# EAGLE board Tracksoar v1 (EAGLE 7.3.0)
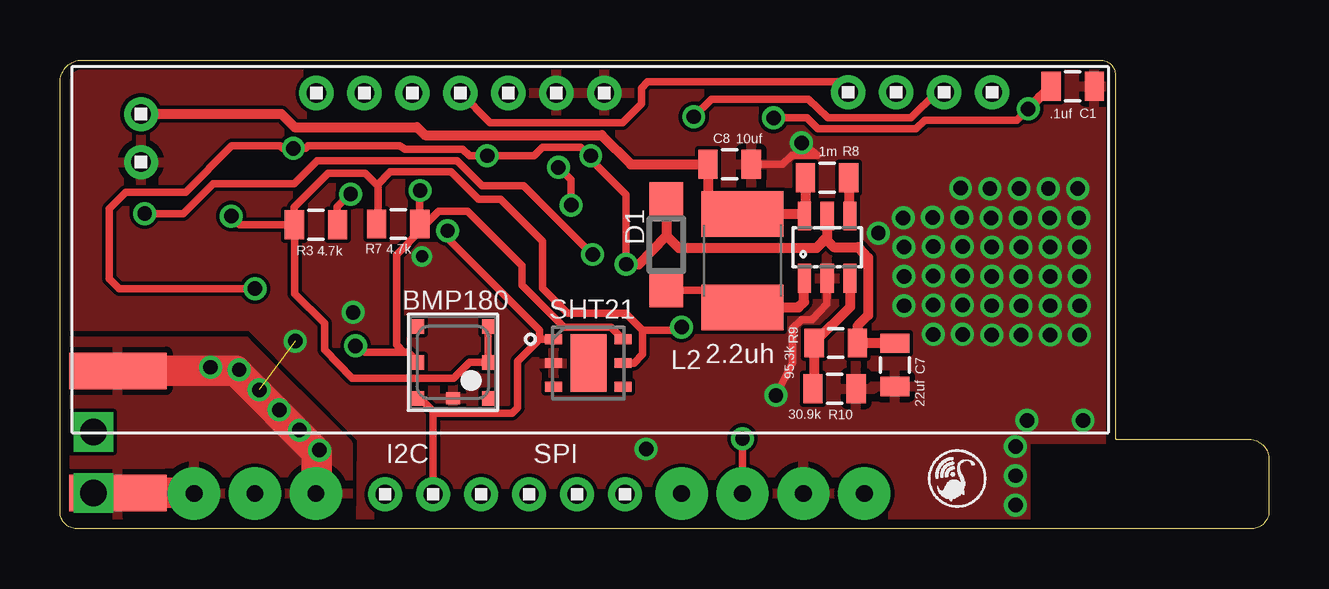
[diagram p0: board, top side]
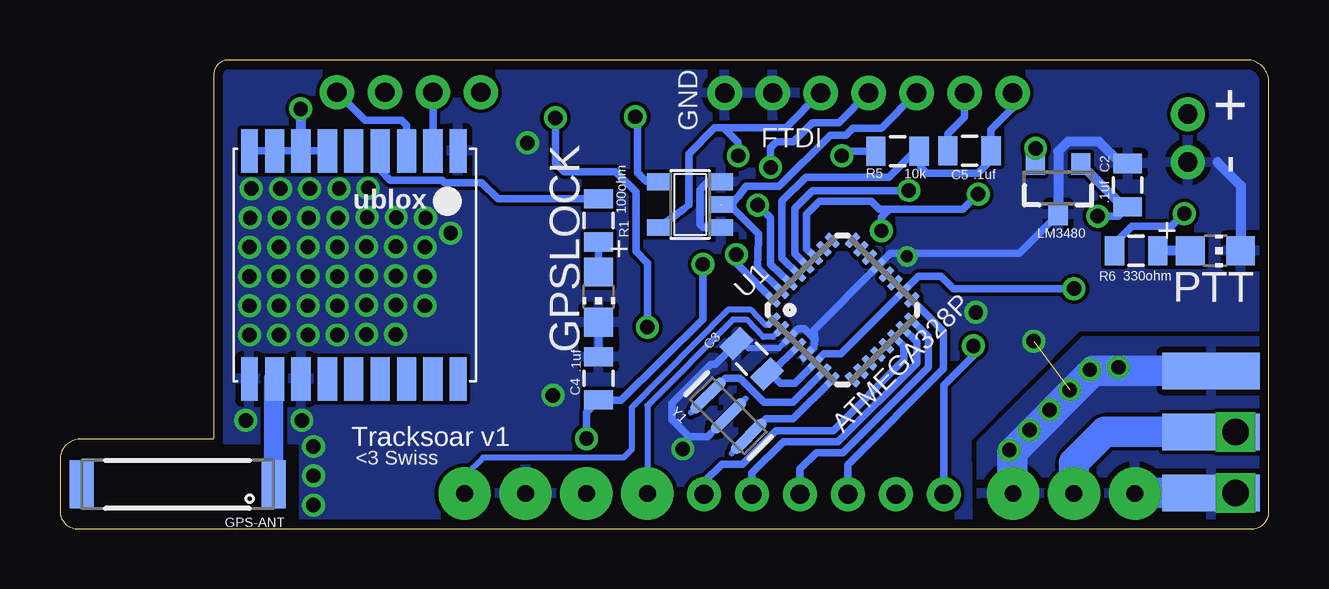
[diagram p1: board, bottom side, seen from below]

Size 50.39 x 19.53 mm. Coordinates in mm from the lower left corner, seen from the top.
Outline: 0.69,0 arc-90 0,0.76 0,18.67 arc-90 0.99,19.53 43.38,19.53 arc-90 43.99,18.87 43.99,3.78 arc90 44.04,3.73 49.58,3.73 arc-90 50.39,2.87 50.39,0.79 arc-90 49.68,0 0.69,0
Copper layers (1*16): Top 0.0356mm / dielectric 1.5011mm / Bottom 0.0356mm
Design rules "oshpark-2layer": minimum track width 6mil, minimum drill 13mil, track to track 6mil, track to pad 6mil, pad to pad 6mil, via to via 6mil, smd to smd 6mil, copper to edge 15mil, drill to drill 6mil, minimum pad ring 7mil, minimum via ring 7mil, stop-mask expansion 4mil, vias tented up to drill 0mil, thermal gap 10mil

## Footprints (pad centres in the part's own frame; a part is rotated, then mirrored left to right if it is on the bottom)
BMP180 = smd 0.6 x 0.5: 1 1.5,1.45; 2 0,1.45; 3 -1.5,1.45; 4 -1.5,-1.45; 5 0,-1.45; 6 1.5,-1.45 | smd 0.5 x 0.6: 7 1.5,0
0805 = smd 0.8 x 1.2: 1 -0.9,0; 2 0.9,0
SOD123 = smd 1.4 x 1.4: A 1.9,0; C -1.9,0
1X7 = drill 0.8 pad 1.422: 1 -6,0; 2 -4,0; 3 -2,0; 4 0,0; 5 2,0; 6 4,0; 7 6,0
ANTENNA-CHIP4 = smd 1 x 2: NC 4,0; SIG -4,0
CHIP-LED0805 = smd 1.2 x 1.2: A 0,-1.05; C 0,1.05
SOT23-5 = smd 0.69 x 0.99: 1 -0.95,-1.29; 2 0,-1.29; 3 0.95,-1.29; 4 0.95,1.3; 5 -0.95,1.3
SMA-EDGE = smd 1.524 x 4.064: GND@0 0,0; GND@1 5.08,0; SIG 2.54,0 | smd 1.524 x 4.064 bottom: GND@2 0,0; GND@3 5.08,0
L1812 = smd 1.9 x 3.4: 1 -1.95,0; 2 1.95,0
SOT23-3 = smd 0.8 x 0.9: 1 -0.95,-1; 2 0.95,-1; 3 0,1.1
SOT23-6 = smd 0.55 x 1.2: 1 -0.95,-1.3; 2 0,-1.3; 3 0.95,-1.3; 4 0.95,1.3; 5 0,1.3; 6 -0.95,1.3
1X4 = drill 0.8 pad 1.422: 1 -3,0; 2 -1,0; 3 1,0; 4 3,0
DFN300X300X110-7N = smd 0.711 x 0.406: 1 -1.448,0.991; 2 -1.448,0; 3 -1.448,-0.991; 4 1.448,-0.991; 5 1.448,0; 6 1.448,0.991 | smd 1.499 x 2.388: 7 0,0
1X6 = drill 0.8 pad 1.422: 1 -5,0; 2 -3,0; 3 -1,0; 4 1,0; 5 3,0; 6 5,0
MLF32 = smd 0.7 x 0.3: 1 -2.35,1.75; 2 -2.35,1.25; 3 -2.35,0.75; 4 -2.35,0.25; 5 -2.35,-0.25; 6 -2.35,-0.75; 7 -2.35,-1.25; 8 -2.35,-1.75; 17 2.35,-1.75; 18 2.35,-1.25; 19 2.35,-0.75; 20 2.35,-0.25; 21 2.35,0.25; 22 2.35,0.75; 23 2.35,1.25; 24 2.35,1.75 | smd 0.3 x 0.7: 9 -1.75,-2.35; 10 -1.25,-2.35; 11 -0.75,-2.35; 12 -0.25,-2.35; 13 0.25,-2.35; 14 0.75,-2.35; 15 1.25,-2.35; 16 1.75,-2.35; 25 1.75,2.35; 26 1.25,2.35; 27 0.75,2.35; 28 0.25,2.35; 29 -0.25,2.35; 30 -0.75,2.35; 31 -1.25,2.35; 32 -1.75,2.35
UBLOX_MAX = smd 1.8 x 0.7: 1_GND 4.95,-4.4; 9_V_RESET 4.95,4.3; 10_GND -4.55,4.3; 18_RESERVED -4.55,-4.4 | smd 1.8 x 0.8: 2_TXD1 4.95,-3.35; 3_RXD1 4.95,-2.25; 4_TIMEPULSE 4.95,-1.15; 5_EXTINT0 4.95,-0.05; 6_V_BCKP 4.95,1.05; 7_VCC_IO 4.95,2.15; 8_VCC 4.95,3.25; 11_RF_IN -4.55,3.25; 12_GND -4.55,2.15; 13_ANTON -4.55,1.05; 14_VCC_RF -4.55,-0.05; 15_RESERVED -4.55,-1.15; 16_SDA2 -4.55,-2.25; 17_SCL2 -4.55,-3.35
RADIOMETRIX-HX1 = drill 0.7 pad 2.184: 0V 8.89,-10.16; EN 3.81,-10.16; RFGND -11.43,-10.16; RFGND2 -16.51,-10.16; RFOUT -13.97,-10.16; TXD 11.43,-10.16; VCC 6.35,-10.16
1X2 = drill 0.8 pad 1.422: 1 -1,0; 2 1,0
RESONATOR-SMD = smd 0.45 x 1.905: 1 -1.2,0; 2 0,0; 3 1.2,0

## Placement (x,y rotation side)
BMP180  BMP180  [BMP180]  16.38,6.93 270 top
C1  .1uf  [0805]  42.22,18.44 180 top
C2  .1uf  [0805]  5.89,14.33 270 bottom
C3  .1uf  [0805]  21.57,7.09 315 bottom
C4  .1uf  [0805]  27.94,6.27 270 bottom
C5  .1uf  [0805]  12.48,15.76 0 bottom
C7  22uf  [0805]  34.8,6.83 270 top
C8  10uf  [0805]  27.92,15.19 0 top
D1  MBR120VLSFT1  [SOD123]  25.27,11.84 270 top
FRAME1  FRAME-LETTER  [CREATIVE_COMMONS]  not placed on the board
FTDI  1X7  [1X7]  16.69,18.16 180 top
GPS-ANT  ANTENNA2SMD3  [ANTENNA-CHIP4]  45.49,1.85 180 bottom
GPSLOCK  [CHIP-LED0805]  27.94,9.65 180 bottom
IC2  74AHC1G125DBV  [SOT23-5]  24.13,13.51 90 bottom
J$1  SMA_EDGE  [SMA-EDGE]  2.41,1.5 90 bottom
L2  2.2uh  [L1812]  28.45,11.18 270 top
LM3480  LM3480IM4  [SOT23-3]  8.79,14.2 180 bottom
LT3426  LT3426  [SOT23-6]  31.98,11.73 0 top
PTT  [CHIP-LED0805]  2.24,11.58 270 bottom
R1  100ohm  [0805]  27.94,12.85 270 bottom
R3  4.7k  [0805]  10.67,12.67 0 top
R5  10k  [0805]  15.48,15.74 180 bottom
R6  330ohm  [0805]  5.54,11.58 180 bottom
R7  4.7k  [0805]  14.1,12.7 0 top
R8  1m  [0805]  31.98,14.63 180 top
R9  95.3k  [0805]  32.33,7.75 0 top
R10  30.9k  [0805]  32.28,5.84 180 top
SERIAL  1X4  [1X4]  35.86,18.19 180 top
SHT21  SHT21  [DFN300X300X110-7N]  22.02,6.91 0 top
SPI/I2C  1X6  [1X6]  18.56,1.43 0 top
U1  ATMEGA328P  [MLF32]  17.78,9.12 45 bottom
U$1  UBLOX_MAX  [UBLOX_MAX]  38.2,10.79 90 bottom
U$2  RADIOMETRIX-HX1  [RADIOMETRIX-HX1]  22.1,11.63 0 top
U$3  1X2  [1X2]  3.38,16.28 90 top
Y1  16MHZ  [RESONATOR-SMD]  22.53,4.71 315 bottom

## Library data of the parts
BMP180 = SparkFun-Sensors
C1-C5 C7 C8 = SparkFun-Capacitors
D1 = diode
FRAME1 = SparkFun-Aesthetics
FTDI SERIAL SPI/I2C U$3 = headers(2mm)
GPS-ANT = SparkFun-RF
GPSLOCK LT3426 PTT = adafruit
IC2 = 74xx-little-us
J$1 = SparkFun-Connectors
L2 = resistor
LM3480 = SparkFun-PowerIC
R1 R3 R5-R10 = SparkFun-Resistors
SHT21 = sht21; MPN: SHT21; OC_FARNELL: 1855468; OC_NEWARK: 20T1172; PACKAGE: DFN-6; SUPPLIER: SENSIRION
U1 = SparkFun-DigitalIC
U$1 U$2 = Ava
Y1 = SparkFun-FreqCtrl; PROD_ID: XTAL-08900

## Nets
3V: BMP180.2 BMP180.3 C1.2 C2.2 LM3480.1 R3.1 R7.1 SHT21.5 U$1.6_V_BCKP U$1.7_VCC_IO U$1.8_VCC U$1.9_V_RESET
15V: C8.1 L2.1 LT3426.6 R8.2 U$3.2
!RESET: C5.2 FTDI.7 R5.1 U1.29
D3: U1.1 U$2.TXD
D4: U1.2 U$2.EN
DTR: C5.1 FTDI.6
GND: BMP180.7 C1.1 C2.1 C3.1 C4.1 C7.2 C8.2 FTDI.1 FTDI.2 GPSLOCK.C IC2.1 IC2.3 J$1.GND@0 J$1.GND@1 J$1.GND@2 J$1.GND@3 LM3480.3 LT3426.2 PTT.C R10.1 SHT21.2 U1.3 U1.5 U1.21 U$1.1_GND U$1.10_GND U$1.12_GND U$2.0V U$2.RFGND U$2.RFGND2 U$3.1 Y1.2
LED: R6.2 U1.32
MISO: SPI/I2C.4 U1.16
MOSI: SPI/I2C.5 U1.15
N$1: J$1.SIG U$2.RFOUT
N$3: GPSLOCK.A R1.2
N$6: GPS-ANT.SIG U$1.11_RF_IN
N$9: D1.A L2.2 LT3426.1
N$12: LT3426.4 R8.1
N$13: LT3426.3 R9.1 R10.2
N$14: U1.8 Y1.3
N$26: U1.7 Y1.1
N$27: PTT.A R6.1
PPS: R1.1 U$1.4_TIMEPULSE
RX1: SERIAL.1 U$1.3_RXD1
RXO: FTDI.4 SERIAL.4 U1.30
SCK: SPI/I2C.3 U1.17
SCL: BMP180.5 R7.2 SHT21.6 SPI/I2C.1 U1.28
SDA: BMP180.6 R3.2 SHT21.1 SPI/I2C.2 U1.27
SS: SPI/I2C.6 U1.14
TX: SERIAL.3 U$1.2_TXD1
TX1: IC2.4 SERIAL.2
TXO: FTDI.5 IC2.2 U1.31
VCC: C3.2 C4.2 C7.1 D1.C FTDI.3 IC2.5 LM3480.2 LT3426.5 R5.2 R9.2 U1.4 U1.6 U1.18 U$2.VCC

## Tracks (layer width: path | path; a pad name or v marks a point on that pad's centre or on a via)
3V  (via drill 0.6)
  Top 0.305: R3.1 7.49,12.67 v7.14,13.03 | R3.1 9.77,13.4 11.18,14.81 12.73,14.81 13.21,14.33 | 13.21,14.33 13.26,14.21 13.26,12.76 R7.1 | 13.21,14.33 13.77,14.88 16.31,14.88 17.45,13.74 18.37,13.74 20.12,11.99 20.12,10.03 21.16,8.99 23.57,8.99 24.28,8.28 | R3.1 9.78,12.66 9.78,9.8 11.02,8.56 11.02,7.47 12.17,6.27 16.41,6.27 17.07,6.93 BMP180.2 BMP180.3 | SHT21.5 23.93,6.91 24.28,7.26 24.28,8.28 | 40.89,17.99 C1.2 | 24.28,8.28 25.78,8.28 v25.91,8.41 | v40.36,17.5 39.88,17.02 36.04,17.02 35.69,16.66 31.6,16.66 31.14,17.12 v29.74,17.12
  Top 0.406: C1.2 40.84,17.98 v40.36,17.5
  Bottom 0.305: U$1.9_V_RESET U$1.8_VCC U$1.7_VCC_IO U$1.6_V_BCKP 39.27,15.73 | v7.14,13.03 6.29,13.03 C2.2 | v25.91,8.41 25.91,11.07 26.39,11.56 26.39,14.05 27.23,14.88 29.39,14.88 29.74,15.24 v29.74,17.12
  Bottom 0.406: C2.2 6.07,13.43 LM3480.1 | v40.36,17.5 U$1.7_VCC_IO
15V
  Top 0.406: U$3.2 9.24,17.28 9.78,16.74 14.89,16.74 15.22,16.41 22.58,16.41 23.8,15.19 C8.1 27.02,13.85 27.76,13.11 28.43,13.11 L2.1 30.94,13.13 LT3426.6 31.08,13.08 R8.2
!RESET
  Bottom 0.305: U1.29 20.3,11.28 20.3,13.67 19.3,14.66 15.85,14.66 14.77,15.74 R5.1 14.5,15.06 14.25,14.81 12.14,14.81 11.58,15.37 C5.2 11.58,16.64 10.69,17.53 FTDI.7
D3
  Bottom 0.254: U1.1 20.89,8.48 20.98,8.48 21.59,9.12 22.56,9.12 26.57,5.05 26.57,3.3 26.9,2.97 32.77,2.97 33.53,2.21 U$2.TXD
D4
  Bottom 0.254: U1.2 20.67,8 21.08,8 21.77,8.71 22.35,8.71 25.91,5.13 U$2.EN
DTR
  Bottom 0.305: FTDI.6 12.69,17.16 13.39,16.46 13.39,15.77
  Bottom 0.406: 13.39,15.77 C5.1
GND  (via drill 0.5, 0.6, 1.1)  (1 unrouted)
  Top 0.305: LT3426.2 31.98,9.37 31.34,8.71 30.91,8.71 30.53,8.36 30.53,6.91 v29.85,5.56 | C8.2 30.13,15.19 30.51,15.57 31.57,15.57 v30.91,16.08
  Top 0.406: U$2.RFGND2 5.61,1.47 5.61,1.5
  Top 1.27: J$1.GND@1 7.32,6.58 10.69,3.2 10.69,1.5 U$2.RFGND | 2.31,1.5 5.61,1.5
  Bottom 0.254: U1.3 20.44,7.52 21.69,7.52 21.9,7.72 C3.1
  Bottom 0.305: U1.5 18.97,7.57 18.92,7.9 | 18.92,7.9 19.36,8.33 19.63,8.33 U1.3 | 18.92,7.9 18.97,8.28 U1.21 15.77,11.48 10.41,11.48 LM3480.3 | GPSLOCK.C C4.1 | 22.85,14.49 IC2.3 22.85,14.45 23.39,14.45 23.72,14.12 23.72,12.7 23.59,12.56 IC2.1 | C3.1 23.07,6.86 23.27,6.86 24.89,5.23 24.89,4.55 24.18,3.84 23.41,3.84 23.25,3.99
  Bottom 0.406: 2.15,15.28 1.17,14.3 1.17,11.6 PTT.C | 5.84,15.28 C2.1 6.18,15.23 7.09,16.13 8.38,16.13 8.79,15.72 LM3480.3
  Bottom 1.27: U$2.RFGND2 5.56,1.5 J$1.GND@2 | J$1.GND@1 7.32,6.58 10.69,3.2 10.69,1.5 U$2.RFGND
  other vias: 9.8,7.82 15.09,11.35 12.22,9.02 1.4,1.5 24.44,3.33 42.49,8.08 41.28,8.08 40.06,8.08 38.84,8.08 37.62,8.1 36.4,8.1 42.49,9.3 41.28,9.3 40.06,9.3 38.84,9.3 37.62,9.32 36.4,9.32 35.18,9.3 42.49,10.52 41.28,10.52 40.06,10.52 38.84,10.52 37.62,10.54 36.4,10.54 35.18,10.52 42.49,11.73 41.28,11.73 40.06,11.73 38.84,11.73 37.62,11.76 36.4,11.76 35.18,11.73 42.47,12.95 41.25,12.95 40.03,12.95 38.81,12.95 41.2,14.17 42.65,4.52 39.83,3.43 39.83,2.21 39.83,0.99 40.31,4.52 39.98,14.17 42.42,14.17 37.59,12.98 36.37,12.98 35.15,12.95 34.11,12.32 38.76,14.17 37.54,14.2 6.27,6.73 7.47,6.63 8.31,5.79 9.14,4.95 9.98,4.11 10.82,3.28
  pour Top: 0,19.56 44.02,19.56 44.02,3.73 40.23,3.73 40.23,0 12.55,0 12.6,3.76 7.95,8.43 0,8.43
  pour Bottom: 0,19.56 44.02,19.56 44.02,3.73 40.23,3.73 40.23,0 12.55,0 12.6,3.76 7.95,8.43 0,8.43
  pour Bottom: 0,7.82 7.72,7.82 11.99,3.56 11.99,0 0,0
  pour Top: 0,7.82 7.72,7.82 11.99,3.56 11.99,0 0,0
LED  (via drill 0.6)
  Top 0.305: v3.53,13.13 5.13,13.13 6.38,14.38 9.75,14.38 10.72,15.34 16.56,15.34 17.6,14.3 19.33,14.3 v22.2,11.43
  Bottom 0.305: R6.2 6.44,11.88 5.72,12.6 4.06,12.6 v3.53,13.13 | v22.2,11.43 22.2,11.06 U1.32
MISO
  Bottom 0.305: U1.16 14.2,8.01 14.2,6.73 17.76,3.17 18.87,3.17 19.55,2.5 SPI/I2C.4
MOSI
  Bottom 0.305: U1.15 14.68,7.79 14.68,6.91 17.96,3.63 20.24,3.63 21.55,2.33 SPI/I2C.5
N$1
  Bottom 1.27: J$1.SIG 6.83,4.04 8.13,2.74 U$2.RFOUT
N$3
  Bottom 0.305: R1.2 GPSLOCK.A
N$6
  Bottom 0.813: U$1.11_RF_IN 41.49,6.24 GPS-ANT.SIG
N$9
  Top 0.305: D1.A 27.74,9.94 L2.2
  Top 0.406: L2.2 30.79,9.23 31.01,9.45 31.01,10.42 LT3426.1
N$12
  Top 0.406: R8.1 32.88,13.08 LT3426.4
N$13
  Top 0.406: LT3426.3 32.93,9.24 R9.1 31.44,5.89 R10.2
N$14
  Bottom 0.305: U1.8 19.85,4.58 20.97,4.58
N$18  (via drill 1.1)
  other vias: 1.4,4.04
N$26
  Bottom 0.305: U1.7 19.85,5.28 21.06,5.28 22.05,6.28 22.66,6.28
N$27
  Bottom 0.406: PTT.A R6.1
PPS
  Bottom 0.305: R1.1 32.14,13.75 32.82,14.43 34.37,14.43 34.47,14.53 36.63,14.53 37.06,14.96 U$1.4_TIMEPULSE
RX1
  Bottom 0.305: U$1.3_RXD1 35.95,16.83 36.15,17.02 37.67,17.02 SERIAL.1
RXO  (via drill 0.6)
  Top 0.305: v21.31,13.49 21.31,14.55 v20.78,15.06 | FTDI.4 17.93,16.92 23.45,16.92 24.23,17.7 24.23,18.36 24.49,18.62 32.43,18.62 SERIAL.4 32.86,18.21
  Bottom 0.305: U1.30 20.78,11.03 20.78,12.95 v21.31,13.49 | v20.78,15.06 20.78,15.87 20.52,16.13 19.81,16.13 19.03,16.92 17.93,16.92 FTDI.4
SCK
  Bottom 0.305: U1.17 13.56,8.23 13.56,6.68 17.55,2.67 SPI/I2C.3
SCL  (via drill 0.6)
  Top 0.305: R7.2 15,13.6 v15.01,14.1 | SHT21.6 22.96,8.41 21.01,8.41 19.27,10.15 U1.28 16.99,13.23 15.77,13.23 15.24,12.7 R7.2 | v12.32,7.62 12.47,7.62 12.73,7.37 14.33,7.37 | 14.33,7.37 14.5,7.37 BMP180.5 | R7.2 15.07,12.48 14.02,11.43 14.02,7.67 14.33,7.37
  Bottom 0.305: U1.28 19.76,11.45 19.76,13.36 19.03,14.1 v15.01,14.1 | v12.32,7.62 12.32,7.21 13.56,5.98 SPI/I2C.1 | SPI/I2C.1
SDA  (via drill 0.6)
  Top 0.305: v12.12,13.94 12.09,13.94 11.56,13.41 11.56,12.69 R3.2 | BMP180.6 15.16,5.29 15.56,4.89 | 15.56,4.89 15.62,4.83 18.85,4.83 19.08,5.05 19.08,6.98 19.99,7.9 | 19.99,7.9 SHT21.1 | 19.99,7.9 19.99,8.28 16.16,12.12 v16.16,12.42 | SPI/I2C.2 15.56,4.89 | 15.56,4.89
  Bottom 0.305: U1.27 19.28,11.68 19.28,13.11 18.75,13.64 16.56,13.64 16.23,13.31 15.83,13.31 | 15.83,13.31 12.75,13.31 v12.12,13.94 | v16.16,12.42 16.16,12.98 15.83,13.31
SS
  Bottom 0.305: U1.14 15.22,7.61 15.22,7.04 18.16,4.09 20.55,4.09 21.95,2.69 22.81,2.69 23.55,1.95 SPI/I2C.6
TX
  Bottom 0.305: U$1.2_TXD1 SERIAL.3
TX1  (via drill 0.6)
  Top 0.305: SERIAL.2 36.56,18.19 35.46,17.12 32,17.12 31.19,17.91 27.15,17.91 v26.42,17.17
  Bottom 0.305: IC2.4 25.89,14.49 25.97,14.49 26.32,14.83 26.32,17.07 v26.42,17.17
TXO
  Bottom 0.305: U1.31 21.31,10.88 21.29,12.09 21.29,12.29 22.35,13.36 | 22.35,13.36 22.66,13.36 IC2.2 | 22.35,13.36 22.35,13.61 22.1,13.87 21.79,14.27 20.42,14.27 18.29,16.41 17.63,16.41 17.35,16.69 16.16,16.69 FTDI.5
VCC  (via drill 0.6)
  Top 0.305: v8.13,10.01 2.46,10.01 2.06,10.41 2.06,13.33 2.74,14.02 5.23,14.02 7.16,15.95 9.17,15.95 9.27,15.85 v9.73,15.85 10.24,15.85 10.34,15.95 14.15,15.95 14.38,15.82 16.79,15.82 17.07,15.54 v17.81,15.54 19.76,15.54 20.12,15.9 21.69,15.9 v22.12,15.54 21.97,15.54 23.6,13.92 v23.6,11.02 | U$2.VCC v28.45,3.76
  Top 0.406: D1.C 25.27,12.22 | 25.27,12.22 25.78,11.71 31.55,11.71 31.98,12.14 LT3426.5 31.98,12.01 32.26,11.73 33.27,11.73 33.68,11.3 33.68,8.89 33.25,8.46 33.25,7.76 R9.2 33.25,7.73 C7.1 | v23.6,11.02 24.13,11.02 25.27,12.22
  Bottom 0.305: U1.4 20.75,6.5 C3.2 20.78,6.48 20.37,6.07 19.77,6.07 U1.6 18.54,7.29 17.84,7.29 U1.18 14.62,10.52 13.67,10.52 13.16,10.01 v8.13,10.01 | IC2.5 24.4,13.32 24.18,13.51 24.18,15.62 23.11,16.71 22.73,16.71 | 22.73,16.71 20.14,16.71 FTDI.3 | v9.73,15.85 9.73,15.21 LM3480.2 | R5.2 17.46,15.74 v17.81,15.54 | v22.12,15.54 22.12,16.1 22.73,16.71 | v28.45,3.76 28.45,4.87 C4.2 | C4.2 27.67,5.37 | v23.6,11.02 23.6,8.74 27,5.36 27.93,5.36 C4.2

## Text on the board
tNames: I2C | SPI
bNames: + | GND | FTDI | - | Tracksoar v1 | <3 Swiss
